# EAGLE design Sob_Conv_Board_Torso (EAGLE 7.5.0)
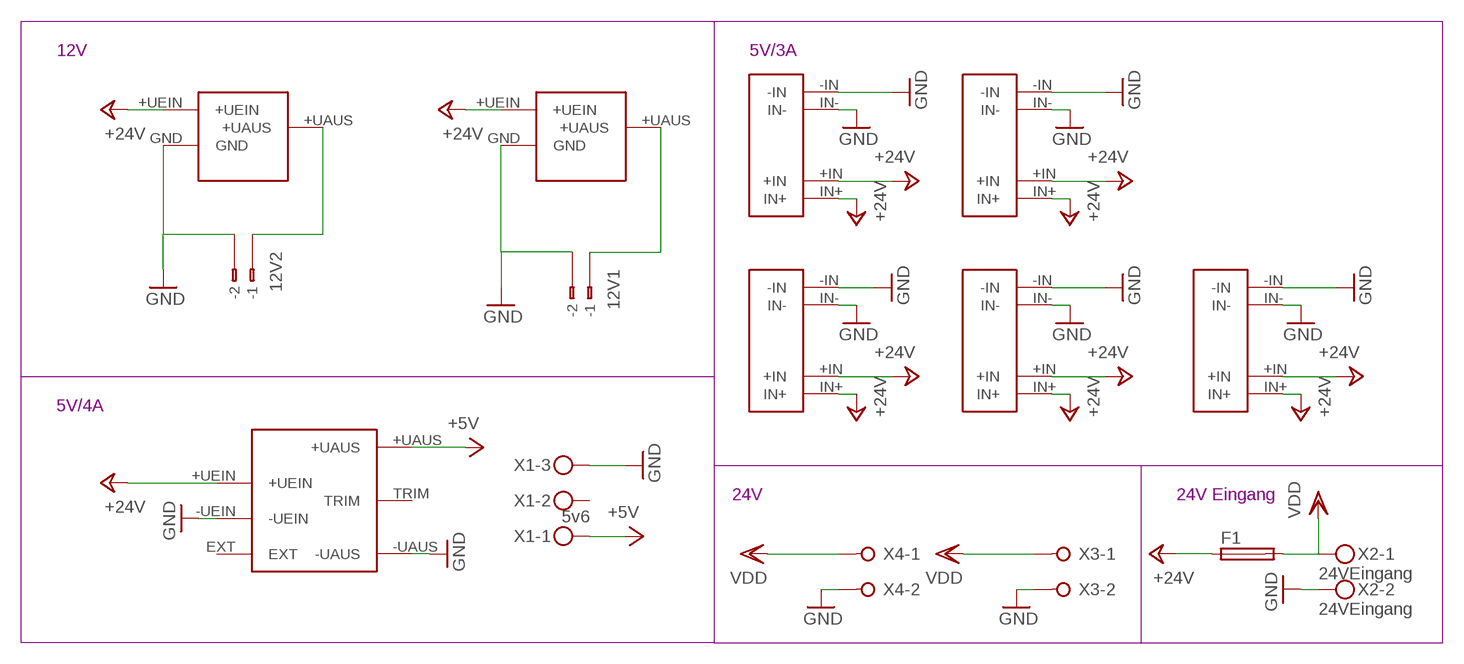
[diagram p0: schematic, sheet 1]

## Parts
12V1  233-102  [233-102]
12V2  233-102  [233-102]
F1  GSH15  [GSH15]
U$1  TEN20-2411WIN  [TEN20-2411WIN]
U$2  TSR1-24120  [TSR1-24120]
U$3  TSR1-24120  [TSR1-24120]
U$4  DCDC25/5V  [DCDC24/5V]
U$5  DCDC25/5V  [DCDC24/5V]
U$6  DCDC25/5V  [DCDC24/5V]
U$7  DCDC25/5V  [DCDC24/5V]
U$8  DCDC25/5V  [DCDC24/5V]
X1  5v6  MKDSN1,5/3-5,08  [MKDSN1,5/3-5,08]
X2  24VEingang  MKDSN1,5/2-5,08  [MKDSN1,5/2-5,08]
X3  W237-02P  [W237-132]
X4  W237-02P  [W237-132]

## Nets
+5V: U$1.+UAUS X1.1
+24V: F1.1 U$1.+UEIN U$2.+UEIN U$3.+UEIN U$4.+IN U$4.IN+ U$5.+IN U$5.IN+ U$6.+IN U$6.IN+ U$7.+IN U$7.IN+ U$8.+IN U$8.IN+
GND: 12V1.B2(B-2) 12V2.B2(B-2) U$1.-UAUS U$1.-UEIN U$2.GND U$3.GND U$4.-IN U$4.IN- U$5.-IN U$5.IN- U$6.-IN U$6.IN- U$7.-IN U$7.IN- U$8.-IN U$8.IN- X1.3 X2.2 X3.2 X4.2
N$1: 12V2.B1(B-1) U$2.+UAUS
N$3: 12V1.B1(B-1) U$3.+UAUS
VDD: F1.2 X2.1 X3.1 X4.1
Unconnected: 12V1.A1(-1) 12V1.A2(-2) 12V2.A1(-1) 12V2.A2(-2) U$1.EXT U$1.TRIM X1.2

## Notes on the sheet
- 12V | 5V/3A
- 5V/4A
- 24V | 24V Eingang

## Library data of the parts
12V1 12V2 = con-wago:233-102: WAGO Cage Clamp; MPN: 233-102; OC_FARNELL: unknown; OC_NEWARK: 28K9044
F1 = fuse:GSH15: FUSE HOLDER; MPN: 64900001039; OC_FARNELL: 1271673; OC_NEWARK: 02P0318
U$1 = ten20-2411win:TEN20-2411WIN
U$2 U$3 = TSR 1-24120:TSR1-24120
U$4-U$8 = dcdc24-5v:DCDC25/5V
X1 = con-phoenix-508:MKDSN1,5/3-5,08: MKDSN 1,5/ 3-5,08 Printklemme Nennstrom: 13,5 A Nennspannung: 250 V Rastermaß: 5,08 mm Polzahl: 3 Anschlussart: Schraubanschluss Montage: Löten Anschlussrichtung Leiter/Platine: 0 ° Artikelnummer: 1729131 Source: http://eshop.phoenixcontact.com .. 1729131.pdf
X2 = con-phoenix-508:MKDSN1,5/2-5,08: MKDSN 1,5/ 2-5,08 Printklemme
X3 X4 = con-wago-508:W237-02P: WAGO SREW CLAMP; OC_FARNELL: unknown; OC_NEWARK: unknown

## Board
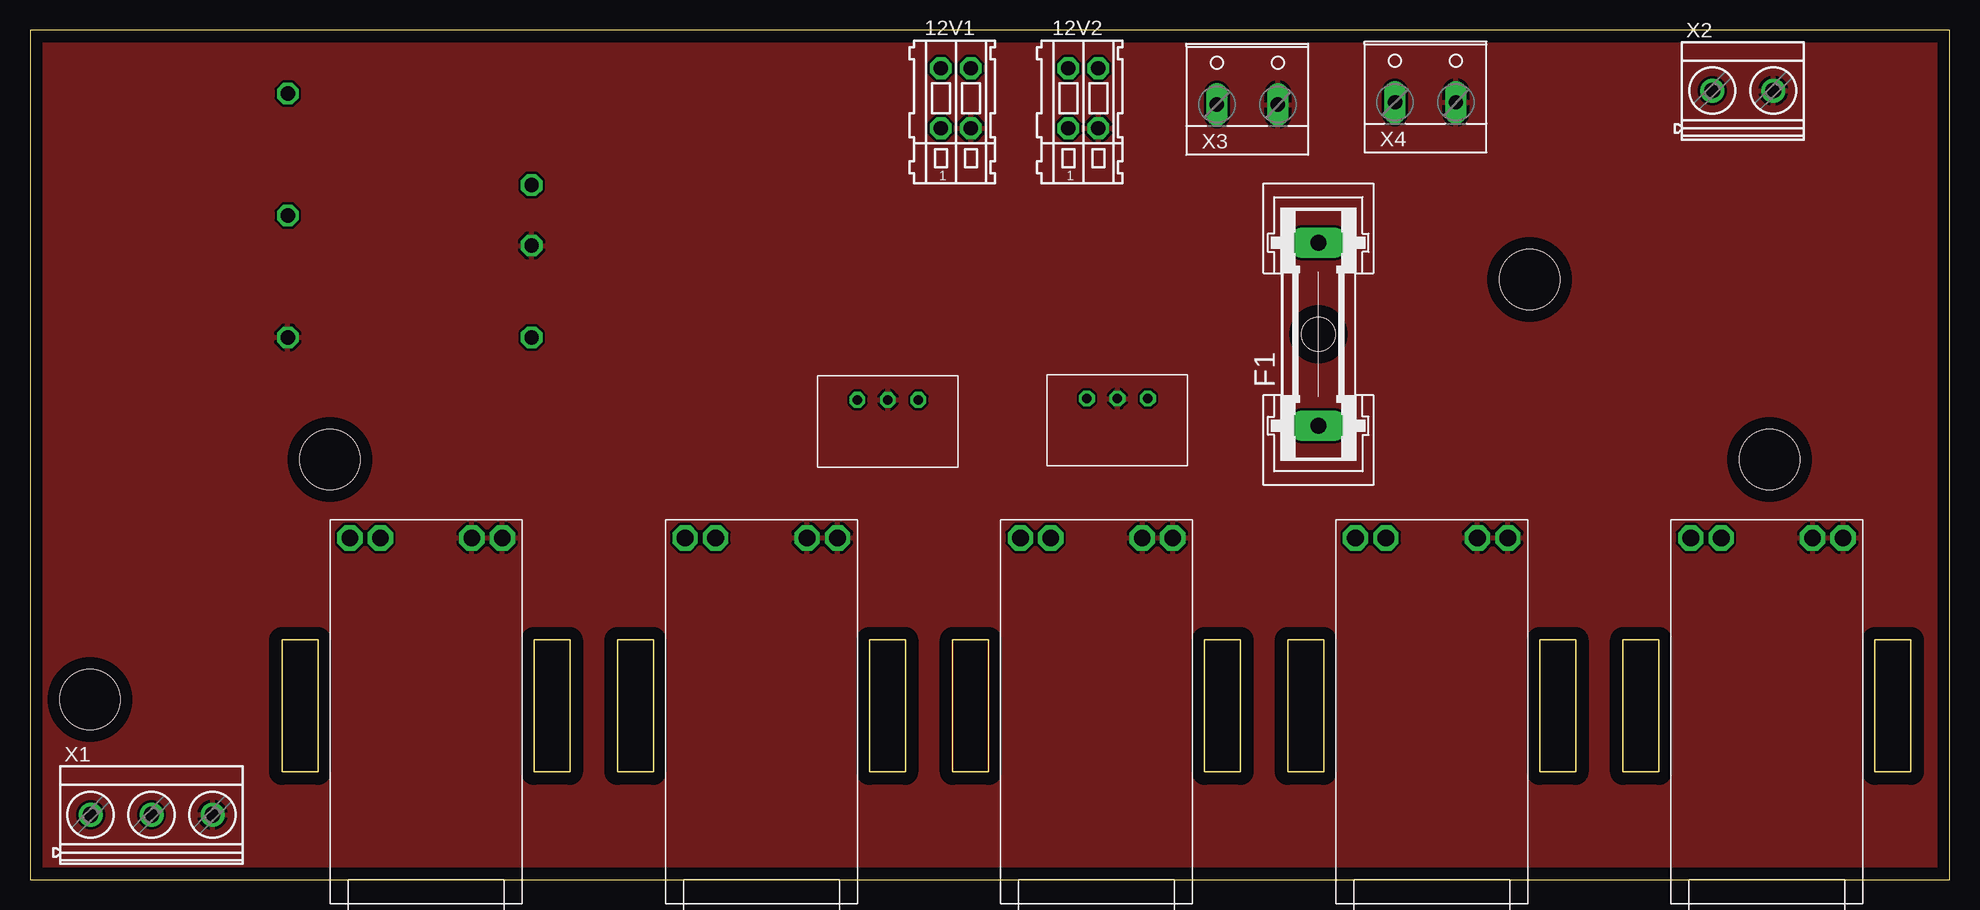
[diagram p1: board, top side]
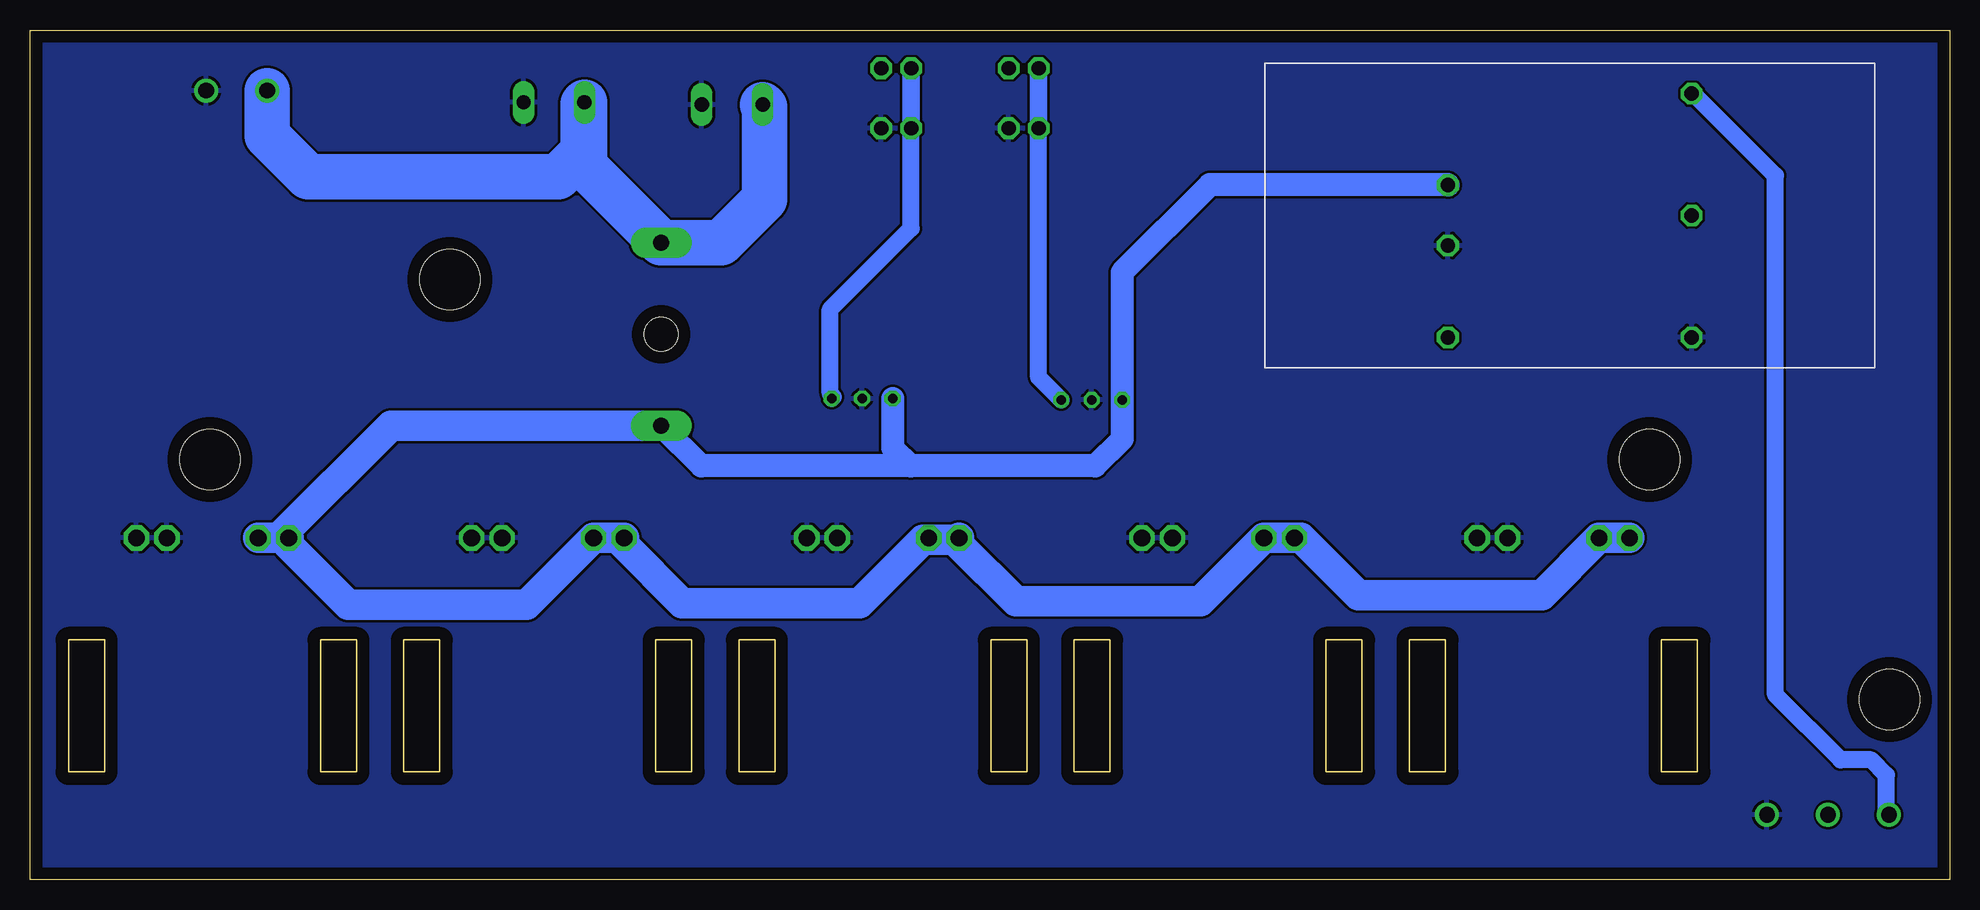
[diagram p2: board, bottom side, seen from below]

Size 160 x 70.8 mm. Coordinates in mm from the lower left corner, seen from the top.
Outline: 0,0 160,0 160,70.8 0,70.8 0,0
Copper layers (1*16): Top 0.035mm / dielectric 1.5mm / Bottom 0.035mm
Design rules "default": minimum track width 10mil, minimum drill 24mil, track to track 8mil, track to pad 8mil, pad to pad 8mil, via to via 8mil, smd to smd 8mil, copper to edge 40mil, drill to drill 8mil, minimum pad ring 10mil, minimum via ring 8mil, stop-mask expansion 4mil, vias tented up to drill 0mil, thermal gap 10mil
Holes 5 mm at 125,50 145,35 5,15 25,35

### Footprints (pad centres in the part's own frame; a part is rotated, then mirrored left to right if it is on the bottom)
233-102 = drill 1.2 octagon: A1 -1.25,2.5; A2 1.25,2.5; B1 -1.25,-2.5; B2 1.25,-2.5
GSH15 = drill 1.321 pad 2.54 long: 1 -7.62,0; 2 7.62,0 | hole 2.794: 0,0
TEN20-2411WIN = drill 1.2 octagon: +UAUS 8.89,-11.43; +UEIN -11.43,-3.81; -UAUS 8.89,8.89; -UEIN -11.43,1.23; EXT -11.43,8.89; TRIM 8.89,-1.27
TSR1-24120 = drill 0.8 octagon: +UAUS 2.54,0; +UEIN -2.54,0; GND 0,0
DCDC24/5V = drill 1.4 octagon: +IN -14.5,-3.81; -IN -14.5,6.35; IN+ -14.5,-6.35; IN- -14.5,3.81
MKDSN1,5/3-5,08 = drill 1.3 pad 2: 1 -7.641,0.025; 2 -2.561,0.025; 3 2.519,0.025
MKDSN1,5/2-5,08 = drill 1.3 pad 2: 1 -2.561,0.025; 2 2.519,0.025
W237-132 = drill 1.194 long: 1 -2.54,-0.635; 2 2.54,-0.635

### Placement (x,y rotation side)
12V1  77.17,65.11 0 top
12V2  87.8,65.11 0 top
F1  107.39,45.45 90 top
U$1  30.38,54.07 180 top
U$2  90.64,40.08 0 top
U$3  71.51,39.98 0 top
U$4  33.02,13.97 270 top
U$5  60.96,13.97 270 top
U$6  88.9,13.97 270 top
U$7  116.84,13.97 270 top
U$8  144.78,13.97 270 top
X1  12.69,5.38 0 top
X2  142.79,65.72 0 top
X3  101.47,65.22 0 top
X4  116.32,65.41 0 top

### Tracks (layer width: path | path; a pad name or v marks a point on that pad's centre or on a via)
+5V
  Bottom 1.422: X1.1 5.25,5.61 5.25,8.71 6.52,9.98 9.07,9.98 14.51,15.42 14.51,58.66 21.35,65.5 U$1.+UAUS
+24V
  Bottom 1.93: U$6.+IN 85.17,28.39 85.17,28.3 | U$1.+UEIN 41.85,57.92 61.65,57.92 68.97,50.6 U$3.+UEIN 68.97,36.71 71.21,34.47 86.58,34.47 | 86.58,34.47 88.07,35.96 88.07,40.05 U$2.+UEIN | 86.58,34.47 104.03,34.47 F1.1
  Bottom 2.54: U$4.IN+ U$4.+IN 34,23.68 49.27,23.68 54.05,28.47 U$5.IN+ U$5.+IN 62.43,23.19 77.82,23.19 82.55,27.92 U$6.IN+ 82.72,28.3 85.17,28.3 85.58,28.3 90.86,23.02 105.63,23.02 110.49,27.89 U$7.IN+ U$7.+IN 118.58,22.91 133.5,22.91 138.43,27.85 U$8.IN+ 139.27,28.47 | 139.27,28.47 U$8.+IN 139.65,28.47 | F1.1 129.91,37.83 139.27,28.47
GND
  pour Bottom: -2.02,71.93 162.66,72.64 160.7,-0.2 -1.36,0.16
  pour Top: -0.6,71.9 162.5,71.9 163.2,-1.1 0.1,-1.1
N$1
  Bottom 1.422: U$2.+UAUS 93.03,40.23 93.3,40.51 93.3,47.52 86.54,54.28 86.54,67.78 86.55,67.77 12V2.B1
N$3
  Bottom 1.422: U$3.+UAUS 75.92,41.85 75.92,67.67 12V1.B1
VDD
  Bottom 3.81: X2.1 140.23,61.99 136.81,58.57 115.98,58.57 113.91,60.64 113.91,64.64 X4.1 113.78,59.46 F1.2 102.38,53.07 98.77,56.68 98.77,64.42 X3.1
